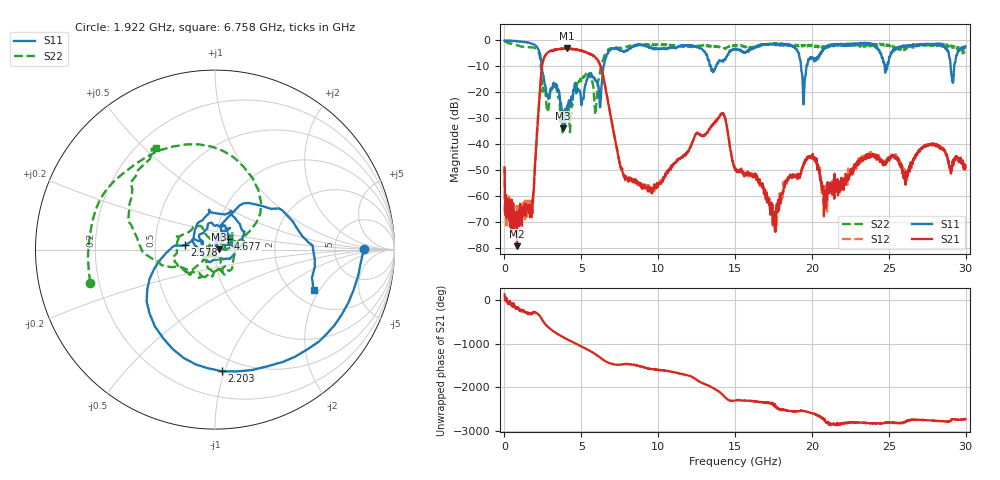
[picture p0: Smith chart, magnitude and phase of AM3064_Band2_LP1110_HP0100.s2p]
# Hz S DB R 50.0
!freq dBS11 angS11 dBS21 angS21 dBS12 angS12 dBS22 angS22
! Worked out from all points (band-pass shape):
!   1600 points, 10 MHz to 29.98 GHz, reference 50 ohm
!   highest |S21| = -3.09 dB at 4.059 GHz (marker M1); lowest = -79.5 dB at 816 MHz (marker M2)
!   |S21| within 3 dB of the highest: 2.629 GHz to 5.827 GHz (3.199 GHz wide, 75.7 % of centre)
!   lowest |S11| = -34.0 dB at 3.815 GHz (marker M3), VSWR 1.04, Z = 52 + j0.0662 ohm
!   |S11| at or under -10 dB: 2.426 GHz to 6.454 GHz (4.028 GHz wide, 90.7 % of centre); 13.43 GHz to 13.77 GHz (346.9 MHz wide, 2.55 % of centre); 19.29 GHz to 19.64 GHz (349.7 MHz wide, 1.8 % of centre)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
!   |S22| runs from -36.4 to -0.2 dB; largest |S21 - S12| = 0.023
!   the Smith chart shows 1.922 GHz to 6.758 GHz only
!   S11 on the Smith chart (normalised r, x): 1.922 GHz: 11, +0; 2.203 GHz: 0.39, -0.98; 2.578 GHz: 0.71, +0.04; 4.677 GHz: 1.15, +0.14; 6.758 GHz: 2.55, -1.77
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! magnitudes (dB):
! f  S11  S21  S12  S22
! 10 MHz  0.0  -49.2  -48.6  -0.2
! 816 MHz  -0.3  -79.5  -68.6  -1.9
! 1.922 GHz  -1.6  -55.7  -55.8  -2.9
! 2.203 GHz  -3.4  -28.1  -28.0  -4.3
! 2.578 GHz  -15.4  -6.7  -6.7  -18.1
! 3.815 GHz  -34.0  -3.2  -3.1  -30.7
! 4.059 GHz  -26.2  -3.1  -3.2  -29.5
! 4.677 GHz  -20.4  -3.5  -3.5  -18.7
! 5.015 GHz  -25.0  -4.0  -3.9  -15.9
! 5.933 GHz  -15.7  -6.6  -6.7  -28.0
! 6.758 GHz  -4.5  -24.5  -24.5  -3.6
! 7.807 GHz  -4.4  -53.2  -52.3  -2.9
! 10 GHz  -3.4  -55.7  -56.0  -1.8
! 14.14 GHz  -7.8  -28.1  -28.4  -2.9
! 15 GHz  -3.3  -50.1  -49.8  -2.0
! 17.59 GHz  -1.3  -73.7  -67.1  -1.1
! 19.47 GHz  -24.0  -47.7  -47.4  -2.3
! 19.99 GHz  -6.4  -44.7  -44.9  -1.8
! 20.83 GHz  -3.3  -64.2  -59.8  -2.4
! 25 GHz  -8.1  -45.4  -46.2  -1.7
! 29.18 GHz  -16.3  -47.3  -46.7  -2.2
! 29.98 GHz  -2.3  -48.8  -48.9  -4.5
